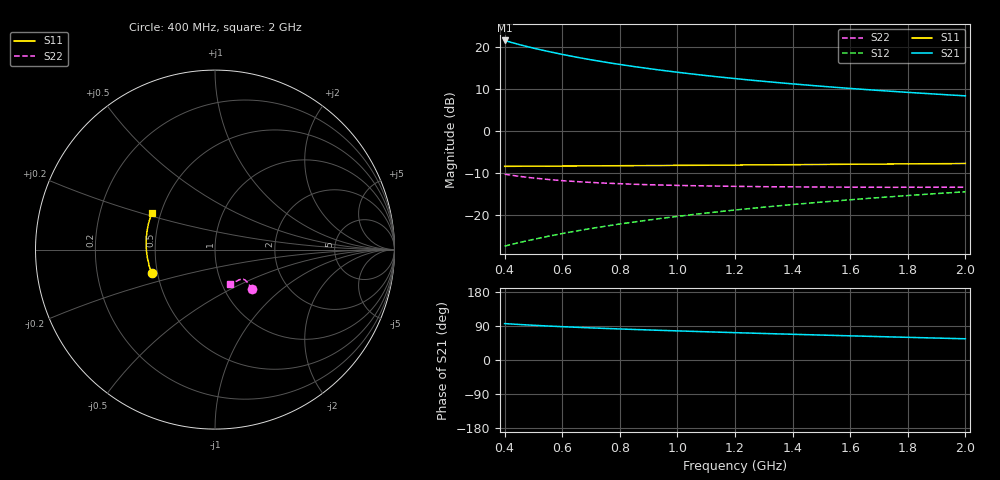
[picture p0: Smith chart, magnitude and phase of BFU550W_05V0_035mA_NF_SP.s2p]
! Filename:  P:\Prog\Test\Noise\ATS_data\Testdata_Net\06 Compressed Noise after Statistics\BFU550W_APM2013_11_D05_05p0V_035mA_NF_CM01_D.sf
! Date/Time: Tue 26/Mar/2013 16:25:23
! BFU550W_APM2013_11_D05_05p0V_1to35mA_NF_CM01_Bias9_R.sf
! Noise Parameter Data File
! BFU550W_APM2013_11_D05_05p0V_1to35mA_NF_CM01
! Date/time: Mon Mar 25 13:26:50 2013
! VAR V_out= 5.000000
! VAR I_out= 35.005000
! VAR V_in= 0.821900
! VAR I_in= 0.373750
! Device data file deembeded for feedlines and parallel
! Original file: \06 Compressed Noise after Statistics\BFU550W_APM2013_11_D05_05p0V_035mA_NF_CM01_R.sf
! Feed-files: PR019V01_070313_Feed1.s2p, PR019V01_070313_Feed2.s2p
! Parallel-file: PR019V01_070313_Par.s2p
# MHz S MA R 50
!  Freq-MHz  S11-mag  S11-arg  S21-mag  S21-arg  S12-mag  S12-arg  S22-mag  S22-arg
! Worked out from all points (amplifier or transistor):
!   37 points, 400 MHz to 2 GHz, reference 50 ohm
!   highest |S21| = 21.5 dB at 400 MHz (marker M1)
!   |S21| within 3 dB of that: start of sweep to 577.7 MHz
!   unconditionally stable (mu >= 1): 756.7 MHz to 1.85 GHz
!   at 500 MHz: K = 0.96, MSG = 22.8 dB, |S12| = -25.9 dB
!   at 1.1 GHz: K = 1.01, MAG = 15.6 dB, |S12| = -19.6 dB
!   at 2 GHz: K = 1.00, MSG = 11.4 dB, |S12| = -14.6 dB
!   lowest NFmin = 1.20 dB at 460 MHz
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400  0.3754 -159.7  11.9 96.1  0.042 70.5  0.3028 -46.6
420  0.3762 -161.2  11.37 95.1  0.04372 70.8  0.2959 -46.5
433  0.3761 -162.3  11.05 94.5  0.04484 71.0  0.2914 -46.3
460  0.3771 -164.0  10.44 93.3  0.04715 71.4  0.2831 -46.1
500  0.3782 -166.7  9.644 91.6  0.05056 71.8  0.2728 -45.8
550  0.3769 -169.5  8.825 89.7  0.055 72.3  0.2625 -45.5
600  0.3792 -172.0  8.121 87.9  0.05939 72.7  0.2536 -45.2
650  0.3794 -174.3  7.521 86.3  0.0638 73.0  0.2474 -45.2
700  0.3805 -176.4  7.004 84.8  0.06824 73.2  0.2416 -45.4
750  0.3818 -178.2  6.556 83.3  0.07269 73.3  0.2369 -45.5
800  0.3822 179.8  6.162 81.9  0.07715 73.4  0.2334 -45.9
850  0.3835 178.0  5.814 80.5  0.08159 73.4  0.2297 -46.1
900  0.384 176.6  5.504 79.3  0.0861 73.5  0.227 -46.5
950  0.3844 174.9  5.224 78.0  0.09064 73.4  0.2247 -47.0
1050  0.3867 172.1  4.748 75.6  0.09971 73.2  0.2211 -48.1
1150  0.3895 169.2  4.352 73.3  0.1087 72.9  0.2182 -49.5
1200  0.3893 168.0  4.183 72.2  0.1134 72.7  0.2171 -50.4
1350  0.3923 164.3  3.741 68.9  0.1271 72.1  0.2142 -52.6
1500  0.3953 160.8  3.388 65.8  0.1409 71.3  0.2132 -55.6
1650  0.3987 157.4  3.101 62.8  0.1547 70.4  0.2122 -58.5
1750  0.4009 155.5  2.939 60.8  0.164 69.7  0.2114 -60.6
2000  0.4068 150.3  2.602 56.0  0.1871 68.0  0.2119 -66.5
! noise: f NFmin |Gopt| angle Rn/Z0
400  1.238  0.4239  -170.9  0.0627
460  1.203  0.4264  -169  0.0672
600  1.275  0.4206  -165.3  0.0706
800  1.298  0.445  -161.9  0.0674
1000  1.327  0.4413  -157.2  0.0766
1200  1.367  0.4571  -153.8  0.0806
1400  1.399  0.4606  -149.3  0.0943
1600  1.442  0.4737  -145.4  0.099
1800  1.473  0.5079  -139.7  0.1094
2000  1.539  0.4946  -137.3  0.1281
